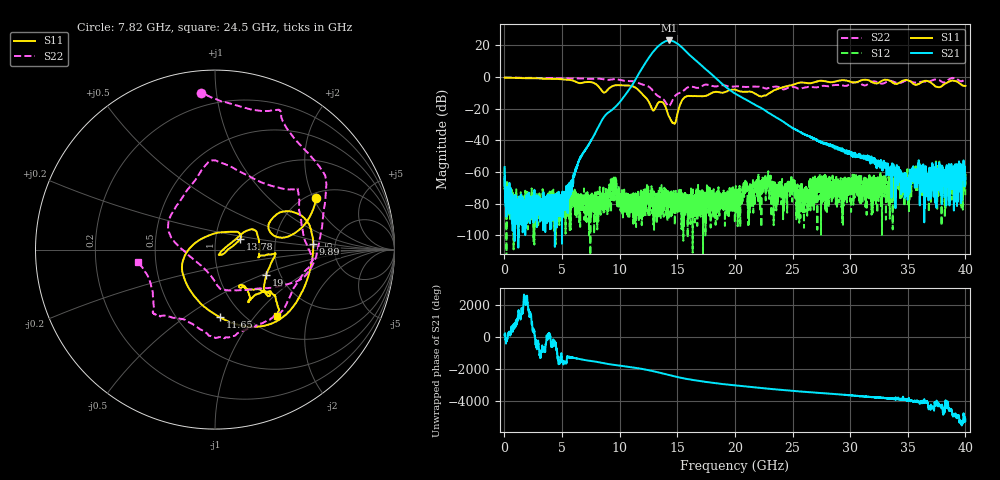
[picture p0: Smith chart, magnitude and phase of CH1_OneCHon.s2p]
!Keysight Technologies,N5245B,MY57181321,A.14.80.03
!Date: Thursday, August 24, 2023 18:38:51
!Correction: S11(C  2-Port  )
!S21(C  2-Port  )
!S12(C  2-Port  )
!S22(C  2-Port  )
!S2P File: Measurements: S11, S21, S12, S22:
# Hz S  RI  R 50
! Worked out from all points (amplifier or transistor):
!   4000 points, 10 MHz to 40 GHz, reference 50 ohm
!   highest |S21| = 23.0 dB at 14.3 GHz (marker M1)
!   |S21| within 3 dB of that: 13.45 GHz to 15.18 GHz (1.732 GHz wide, 12.1 % of centre)
!   unconditionally stable (mu >= 1): start of sweep to end of sweep
!   at 6.67 GHz: K = 175926.24, MAG = -40.4 dB, |S12| = -79.9 dB
!   at 20.01 GHz: K = 3833.16, MAG = -8.5 dB, |S12| = -71.2 dB
!   at 40 GHz: K = 726302.12, MAG = -55.9 dB, |S12| = -74.8 dB
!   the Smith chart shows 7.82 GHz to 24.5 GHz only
!   S11 on the Smith chart (normalised r, x): 7.82 GHz: 2.19, +2.09; 9.89 GHz: 3.40, +0.32; 11.65 GHz: 0.79, -0.69; 13.78 GHz: 1.32, +0.16; 19 GHz: 1.70, -0.53; 24.5 GHz: 1.32, -1.31
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1e7  -0.9473 0.0461  -0.00127 0.000659  0.00134 0.000292  -0.9532 0.0232
6.68e9  0.2952 0.5711  0.00282 0.00145  -0.000145 2.36e-05  -0.3528 0.8246
7.82e9  0.5612 0.2871  -0.00334 -0.0152  -8.84e-05 0.000163  -0.0754 0.8714
9.89e9  0.5475 0.0324  0.1404 0.0231  9.1e-05 0.000106  0.3692 0.7406
1.165e10  0.0278 -0.3775  -1.233 -0.2233  2.66e-05 -2.44e-06  0.6031 0.1922
1.265e10  -0.1303 0.019  3.016 3.583  -9.46e-05 8.22e-05  0.4096 -0.1911
1.304e10  0.0141 0.0941  6.995 -1.595  -3.24e-05 6.13e-05  0.2229 -0.2191
1.334e10  0.1137 0.0998  4.096 -8.345  -0.000116 0.000183  0.0948 -0.2277
1.378e10  0.1406 0.0579  -9.591 -7.757  5.47e-05 9.39e-05  0.0114 -0.1983
1.404e10  0.0975 0.018  -13.53 1.955  -2.48e-05 3.42e-05  -0.0251 -0.1446
1.43e10  0.0503 -0.0219  -7.928 11.78  -4.26e-05 8.32e-05  -0.0928 -0.0759
1.458e10  0.0211 -0.0291  3.92 13.01  0.000125 0.000102  -0.1828 0.00147
1.494e10  0.0518 0.006  11.42 2.305  0.000194 4.57e-05  -0.2592 0.1057
1.542e10  0.1581 0.0949  3.723 -7.58  1.75e-05 1.53e-06  -0.187 0.2826
1.605e10  0.235 0.0862  -4.229 -2.659  -6.06e-05 5.42e-05  -0.0335 0.4902
1.688e10  0.245 -0.0351  -1.214 2.453  -5.67e-05 -1.6e-05  0.2648 0.3721
1.9e10  0.2863 -0.1412  0.0375 -0.5554  6.3e-05 6.46e-06  0.5385 -0.0676
2.001e10  0.3065 -0.2508  -0.2826 -0.0942  -0.000258 -9.57e-05  0.3904 -0.3181
2.45e10  0.3451 -0.3688  -0.0161 -0.028  0.000188 0.000222  -0.4291 -0.069
2.667e10  0.1335 -0.6299  -0.00576 0.0105  -0.000274 -0.000236  -0.3244 0.3492
3.334e10  -0.697 -0.3603  -1.14e-05 0.00099  0.00024 0.000655  0.7307 -0.1011
4e10  -0.0685 0.513  -0.000288 0.000613  0.000146 0.00011  0.3455 -0.797
